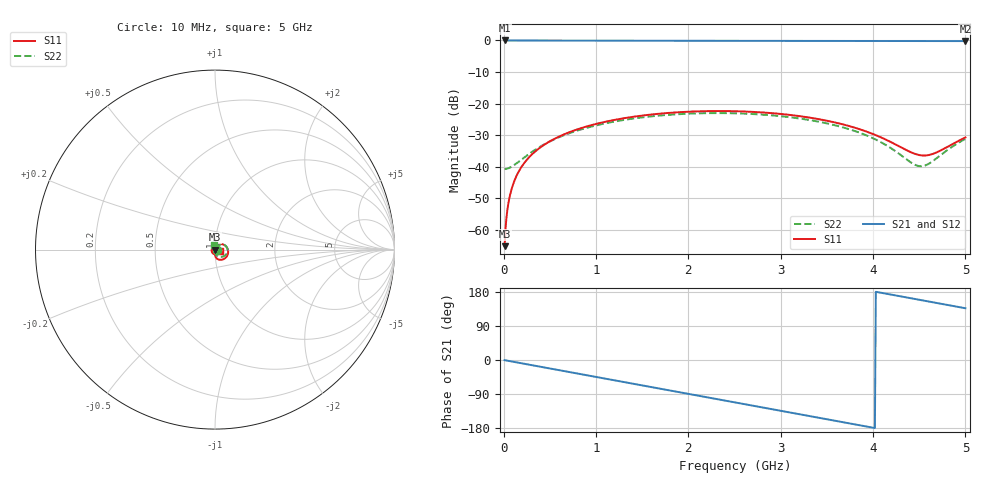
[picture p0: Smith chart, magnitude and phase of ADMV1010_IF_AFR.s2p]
! Analog Devices, Inc.
! 1 Analog Way
! Wilmington, MA 01887
! http://www.analog.com
! Date:  2021-09-07 NN
! Board Name:  ADMV1010-EVALZ Revision B with ADMV1010AEZ installed
! File Description:  Automatic Fixture Removal S-Parameters for IF Port connector and board loss de-embedding
! File Generation:  Calibrated Network Analyzer
! Chip Part Number:  ADMV1010
! Chip Description:  GaAs, MMIC, IQ Downconverter
! Chip Frequency:  12.6 to 15.4 GHz
! Chip Package:  LCC, 4.9 x 4.9 x 1 mm
! IF Port:  ADMV1010AEZ removed and end of trace left open
! Note:
!  Analog Devices supplies this data as a sample of measured data at the evaluation board
!  ports for this product.  Your particular data for this product may vary.
!  Analog Devices reserves the right to change this data at anytime.
!  All lines below in this file are as is from the Network Analyzer.
!Agilent Technologies,N5245A,MY52451809,A.10.47.06
!Automatic Fixture Removal (AFR)
!Date: Thursday, September 09, 2021 11:56:09 PM
!S2P File: Measurements: S11,S21,S12,S22:
# MHz S  RI  R 50
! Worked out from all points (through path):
!   500 points, 10 MHz to 5 GHz, reference 50 ohm
!   highest |S21| = 0.00 dB at 10 MHz (marker M1); lowest = -0.2 dB at 5 GHz (marker M2)
!   group delay of S21, straight-line fit = 124 ps
!   lowest |S11| = -65.2 dB at 10 MHz (marker M3), VSWR 1.00, Z = 50 + j0.0516 ohm
!   |S11| at or under -10 dB: start of sweep to end of sweep
!   |S22| runs from -40.8 to -23.0 dB; largest |S21 - S12| = 1.4e-15
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10  -0.000181 0.000516  1 -0.00782  1 -0.00782  0.0091 0.000415
50  -4.83e-05 0.00258  0.9991 -0.0391  0.9991 -0.0391  0.00917 0.00207
80  0.000143 0.00411  0.9977 -0.0625  0.9977 -0.0625  0.00929 0.00331
130  0.000637 0.00664  0.9941 -0.1014  0.9941 -0.1014  0.0096 0.00536
210  0.00188 0.0106  0.9853 -0.1633  0.9853 -0.1633  0.0104 0.00859
320  0.00446 0.0157  0.9669 -0.2471  0.9669 -0.2471  0.0121 0.0128
460  0.00909 0.0214  0.9333 -0.3509  0.9333 -0.3509  0.0152 0.0178
640  0.0169 0.0269  0.8739 -0.4777  0.8739 -0.4777  0.0206 0.023
850  0.0279 0.0303  0.783 -0.6131  0.783 -0.6131  0.0283 0.0273
1280  0.0518 0.0254  0.536 -0.8344  0.536 -0.8344  0.0464 0.0281
1680  0.0684 0.00784  0.2536 -0.9562  0.2536 -0.9562  0.0613 0.0192
2090  0.073 -0.0171  -0.0592 -0.9853  -0.0592 -0.9853  0.0697 0.00281
2510  0.0633 -0.0411  -0.3717 -0.9125  -0.3717 -0.9125  0.0679 -0.0167
2910  0.044 -0.0548  -0.6325 -0.7538  -0.6325 -0.7538  0.0561 -0.0324
3340  0.0207 -0.0552  -0.8442 -0.5036  -0.8442 -0.5036  0.0356 -0.0404
3810  0.00325 -0.0409  -0.9675 -0.1674  -0.9675 -0.1674  0.0109 -0.0346
4170  0.000805 -0.0254  -0.975 0.1074  -0.975 0.1074  -0.0036 -0.0203
4430  0.00537 -0.0155  -0.9324 0.3015  -0.9324 0.3015  -0.00928 -0.00617
4530  0.00836 -0.0125  -0.9057 0.3732  -0.9057 0.3732  -0.0101 -0.000256
4670  0.0134 -0.00928  -0.859 0.4695  -0.859 0.4695  -0.01 0.00818
4850  0.0211 -0.00727  -0.784 0.5847  -0.784 0.5847  -0.00759 0.0189
5000  0.028 -0.00757  -0.7097 0.6718  -0.7097 0.6718  -0.00364 0.0272
